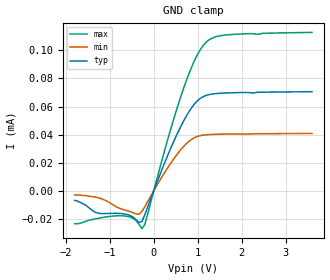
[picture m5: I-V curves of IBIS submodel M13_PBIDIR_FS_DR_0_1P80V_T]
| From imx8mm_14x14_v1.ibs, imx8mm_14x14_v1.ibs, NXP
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| Submodel
[Submodel]  M13_PBIDIR_FS_DR_0_1P80V_T
Submodel_type Dynamic_clamp
[GND Clamp]
| Voltage   I(typ)   I(min)   I(max)
-1.8V     -6.786uA   -2.861uA   -23.36uA
-1.278V   -15.74uA   -4.768uA   -19.67uA
-672.4mV  -16.38uA   -13.51uA   -17.82uA
-470.7mV  -18.65uA   -15.51uA   -19.52uA
-269mV    -21.73uA   -14.69uA   -26.89uA
-201.7mV  -16.95uA   -11.26uA   -23.87uA
310.3mV   24.63uA    16.08uA    35.64uA
682.8mV   49.86uA    31.7uA     73.27uA
993.1mV   64.07uA    38.75uA    96.86uA
1.241V    68.38uA    40.03uA    107.1uA
1.738V    69.77uA    40.5uA     111.2uA
3.6V      70.57uA    40.88uA    112.8uA
